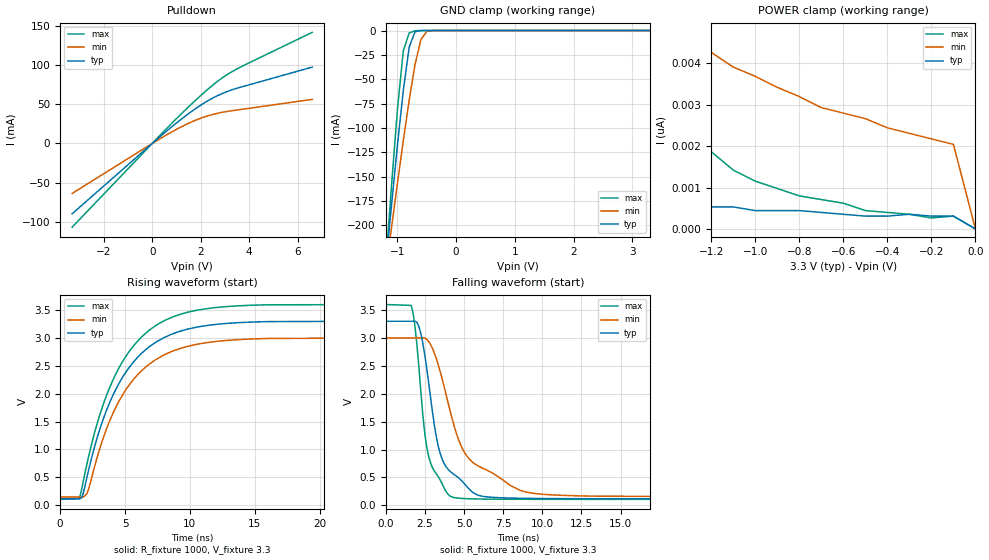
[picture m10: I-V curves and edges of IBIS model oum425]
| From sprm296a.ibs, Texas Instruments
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[Model]   oum425
| PIN IS OUTPUT ONLY BUT MODELLED AS I/O SINCE DRIVER HAS A GZ PIN
Model_type   I/O_open_sink
Enable   Active-Low
Polarity   Non-Inverting
| signals   A, GZ, Y
Vmeas = 1.5
| DUMMY VINH, VINL NEEDED FOR I/O MODEL DESIGNATION
Vinh = 2
Vinl = 0.8
|   typ   min   max
C_comp   3.1345p   2.9748p   5.4957p
|   typ   min   max
[Temperature Range]   25   -40   125
|   typ   min   max
[Voltage Range]   3.30V   3.00V   3.60V
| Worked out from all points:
|   slope of the pulldown table from 0 to 0.495 V, typ, clamps not added: 37.5 ohm
|   GND clamp passes 1 mA (typ) near -0.68 V on its own axis
|   falling waveform, R_fixture 1000, V_fixture 3.3: 20-80 % time 1.21ns typ, 2.37ns min, 832ps max; typ from 3.3 V to 0.117 V
|   rising waveform, R_fixture 1000, V_fixture 3.3: 20-80 % time 3.7ns typ, 3.69ns min, 3.69ns max; typ from 0.117 V to 3.3 V
[Pulldown]
|   Voltage   I(typ)   I(min)   I(max)
-3.3V     -89.53mA   -63.61mA   -106.5mA
600mV     15.94mA    11.1mA     19.19mA
1.5V      37.96mA    25.68mA    46.66mA
2.2V      52.64mA    34.23mA    66.46mA
2.8V      62.35mA    39.14mA    81.55mA
3.4V      69.44mA    42.18mA    93.31mA
6.6V      97.23mA    56.13mA    141.5mA
[GND_clamp]
|   Voltage   I(typ)   I(min)   I(max)
-3.3V     -1.655A    -1.267A    -2.121A
-1.2V     -241.6mA   -247.7mA   -241.2mA
-1.1V     -178.5mA   -201.7mA   -158.3mA
-1V       -117.6mA   -156.6mA   -80.78mA
-900mV    -61.22mA   -112.9mA   -20.65mA
-800mV    -16.98mA   -71.46mA   -2.448mA
-700mV    -1.234mA   -34.72mA   -235.4uA
-600mV    -50.74uA   -9.152mA   -13.23uA
-500mV    -2.357uA   -951.3uA   -456.4nA
-300mV    -4.03nA    -3.368uA   -255.4pA
3.3V      222pA      2.309nA    266.4pA
[POWER_clamp]
|   Voltage   I(typ)   I(min)   I(max)
-3.3V     6.128nA    21.94nA    539.2nA
-3.1V     4.619nA    18.74nA    313.3nA
-2.7V     2.576nA    13.41nA    104.9nA
-2.5V     2.22nA     11.46nA    60.4nA
-2.4V     1.688nA    10.66nA    46.01nA
-1.6V     799.4pA    5.684nA    5.151nA
-1.4V     621.7pA    4.885nA    3.109nA
-1.2V     532.9pA    4.263nA    1.865nA
-1V       444.1pA    3.686nA    1.155nA
-500mV    310.9pA    2.665nA    444.1pA
-100mV    310.9pA    2.043nA    310.9pA
0V        1pA        1pA        1pA
[Ramp]
|   I(typ)   I(min)   I(max)
dV/dt_r   0.001/20n   0.001/30n   0.001/10n
dV/dt_f   1.910/1.208n   1.710/2.366n   2.095/0.824n
[Falling Waveform]
R_fixture = 1000
V_fixture = 3.3
V_fixture_min = 3.0
V_fixture_max = 3.6
|  pd_on
|  TIME   V(typ)   V(min)   V(max)
0s        3.3V       3V         3.6V
1.624ns   3.3V       3V         3.584V
2.119ns   3.204V     3V         2.472V
2.491ns   2.703V     3V         1.296V
2.738ns   2.208V     2.939V     880.6mV
3.357ns   1.058V     2.516V     513.4mV
4.224ns   582.3mV    1.572V     150.6mV
5.462ns   255.6mV    793.8mV    116.9mV
8.929ns   125.5mV    239.8mV    108.7mV
30ns      117.4mV    150.5mV    107.8mV
[Rising Waveform]
R_fixture = 1000
V_fixture = 3.3
V_fixture_min = 3.0
V_fixture_max = 3.6
|  pd_off
|  TIME   V(typ)   V(min)   V(max)
0s        117.4mV    149.9mV    107.8mV
1.477ns   117.4mV    149.9mV    120mV
1.777ns   212mV      149.9mV    426.6mV
2.077ns   515.6mV    213.2mV    753.4mV
3.278ns   1.515V     1.175V     1.775V
4.628ns   2.22V      1.903V     2.499V
6.279ns   2.72V      2.407V     3.013V
8.08ns    3.008V     2.698V     3.31V
13.63ns   3.266V     2.963V     3.568V
30ns      3.298V     2.999V     3.593V
